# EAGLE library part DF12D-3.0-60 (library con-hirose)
60 pin connector PN: DF12D(3.0)-60DP-0.5V Source: con-hirose-df12d(3.0)60dp0.5v80.lbr from Bob Starr <rtzaudio@mindspring.com>
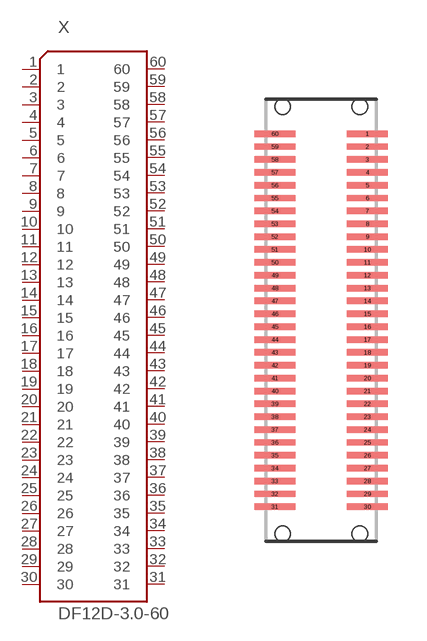
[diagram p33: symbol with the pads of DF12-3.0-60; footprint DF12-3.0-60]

Designator prefix X

## DF12D-3.0-60 (OC_FARNELL: unknown; OC_NEWARK: unknown)  [DF12-3.0-60]
1  1
2  2
3  3
4  4
5  5
6  6
7  7
8  8
9  9
10  10
11  11
12  12
13  13
14  14
15  15
16  16
17  17
18  18
19  19
20  20
21  21
22  22
23  23
24  24
25  25
26  26
27  27
28  28
29  29
30  30
31  31
32  32
33  33
34  34
35  35
36  36
37  37
38  38
39  39
40  40
41  41
42  42
43  43
44  44
45  45
46  46
47  47
48  48
49  49
50  50
51  51
52  52
53  53
54  54
55  55
56  56
57  57
58  58
59  59
60  60

## Footprint DF12-3.0-60 (pad centres in mm)
60 pin connector PN: DF12D(3.0)-60DP-0.5V Hirose Electric Co.
smd 1.6 x 0.25: 1 1.8,7.25; 2 1.8,6.75; 3 1.8,6.25; 4 1.8,5.75; 5 1.8,5.25; 6 1.8,4.75; 7 1.8,4.25; 8 1.8,3.75; 9 1.8,3.25; 10 1.8,2.75; 11 1.8,2.25; 12 1.8,1.75; 13 1.8,1.25; 14 1.8,0.75; 15 1.8,0.25; 16 1.8,-0.25; 17 1.8,-0.75; 18 1.8,-1.25; 19 1.8,-1.75; 20 1.8,-2.25; 21 1.8,-2.75; 22 1.8,-3.25; 23 1.8,-3.75; 24 1.8,-4.25; 25 1.8,-4.75; 26 1.8,-5.25; 27 1.8,-5.75; 28 1.8,-6.25; 29 1.8,-6.75; 30 1.8,-7.25; 31 -1.8,-7.25; 32 -1.8,-6.75; 33 -1.8,-6.25; 34 -1.8,-5.75; 35 -1.8,-5.25; 36 -1.8,-4.75; 37 -1.8,-4.25; 38 -1.8,-3.75; 39 -1.8,-3.25; 40 -1.8,-2.75; 41 -1.8,-2.25; 42 -1.8,-1.75; 43 -1.8,-1.25; 44 -1.8,-0.75; 45 -1.8,-0.25; 46 -1.8,0.25; 47 -1.8,0.75; 48 -1.8,1.25; 49 -1.8,1.75; 50 -1.8,2.25; 51 -1.8,2.75; 52 -1.8,3.25; 53 -1.8,3.75; 54 -1.8,4.25; 55 -1.8,4.75; 56 -1.8,5.25; 57 -1.8,5.75; 58 -1.8,6.25; 59 -1.8,6.75; 60 -1.8,7.25
hole 0.6 at -1.5,8.3
hole 0.6 at 1.5,8.3
hole 0.6 at 1.5,-8.3
hole 0.6 at -1.5,-8.3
